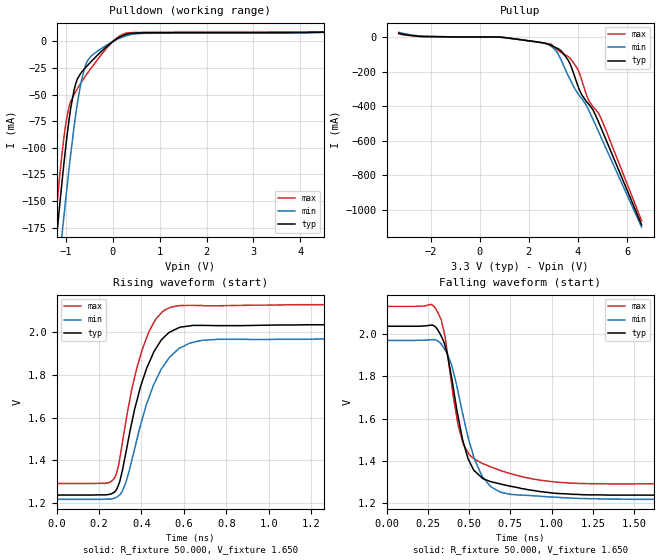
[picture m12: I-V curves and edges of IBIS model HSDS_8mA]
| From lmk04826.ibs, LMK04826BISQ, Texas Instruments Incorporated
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[Model]   HSDS_8mA
Model_type   Output
Polarity   Non-Inverting
Vmeas = 1.9
Vref = 1.9
Cref = 15pF
Rref = 50
|   typ   min   max
|   (nom PVT)   (Fast PVT)   (slow PVT)
C_comp   1.492p   1.392p   1.674p
|C_comp (hi state)   1.492p   1.392p   1.674p
|C_comp (low state)   2.777p   2.419p   2.781p
| Where   nom PVT is  Nominal Process, 3.3V, 27C
|   Fast PVT is Strong Process, 3.45V, -40C
|   Slow PVT is Weak Process, 3.15V, 125C
[Voltage Range]   3.3   3.15   3.45
[Temperature Range]   27   125   -40
[Pullup Reference]   3.3   3.15   3.45
[Pulldown Reference]   0   0   0
[Power Clamp Reference]   3.3   3.15   3.45
[GND Clamp Reference]   0   0   0
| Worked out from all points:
|   slope of the pulldown table from 0 to 0.495 V, typ, clamps not added: 61.7 ohm
|   slope of the pullup table from 0 to 0.495 V, typ, clamps not added: 8 kohm
|   falling waveform, R_fixture 50.000, V_fixture 1.650: 20-80 % time 127ps typ, 150ps min, 119ps max; typ from 2.04 V to 1.24 V
|   rising waveform, R_fixture 50.000, V_fixture 1.650: 20-80 % time 125ps typ, 142ps min, 113ps max; typ from 1.24 V to 2.04 V
[Pulldown]
|   Voltage   I(typ)   I(min)   I(max)
-3.3V     -1.226A    -1.2A      -1.253A
-1.29V    -226.6mA   -272.8mA   -200.2mA
-1.142V   -158.1mA   -207.3mA   -130.7mA
-1.082V   -131.9mA   -181.6mA   -105.5mA
-1.053V   -119.2mA   -168.9mA   -94.06mA
-973.5mV  -87.83mA   -136mA     -69.99mA
-825mV    -45.61mA   -79.95mA   -49.82mA
-686.4mV  -30.15mA   -40.74mA   -39.45mA
-607.2mV  -25.89mA   -25.84mA   -34.12mA
-409.2mV  -16.58mA   -11.85mA   -21.93mA
194.7mV   5.121mA    3.874mA    6.323mA
6.59V     10.59mA    10.66mA    10.59mA
[Pullup]
|   Voltage   I(typ)   I(min)   I(max)
-3.3V     22.42mA    27.3mA     18.86mA
-2.34V    3.185mA    4.961mA    2.641mA
897.6mV   -1.267mA   -2.718mA   -282.3uA
2.363V    -28.99mA   -28.16mA   -29.95mA
2.907V    -48.74mA   -53.27mA   -41.4mA
3.303V    -79.15mA   -129.1mA   -87.94mA
3.679V    -156.2mA   -246.1mA   -122.5mA
3.986V    -278.5mA   -324.2mA   -186mA
4.412V    -384.5mA   -415.9mA   -358.3mA
4.709V    -450mA     -507.1mA   -418.7mA
4.957V    -531.4mA   -585.3mA   -475.6mA
6.59V     -1.086A    -1.1A      -1.063A
[Ramp]
R_load = 50
|   typ   min   max
dV/dt_r   0.471953/1.25144e-10   0.443681/1.42193e-10   0.494567/1.13542e-10
dV/dt_f   0.471995/1.26586e-10   0.443829/1.50046e-10   0.494457/1.19591e-10
[Falling Waveform]
R_fixture = 50.000
V_fixture = 1.650
V_fixture_min = 1.606
V_fixture_max = 1.726
C_fixture = 0.000
|  time   V(typ)   V(min)   V(max)
0s        2.037V     1.97V      2.131V
271.7ps   2.042V     1.973V     2.14V
325.1ps   2V         1.959V     2.078V
354.5ps   1.944V     1.925V     1.989V
392.5ps   1.802V     1.859V     1.774V
466.5ps   1.485V     1.606V     1.476V
578ps     1.32V      1.329V     1.389V
699.3ps   1.289V     1.25V      1.352V
1.17ns    1.241V     1.222V     1.293V
3ns       1.238V     1.218V     1.292V
[Rising Waveform]
R_fixture = 50.000
V_fixture = 1.650
V_fixture_min = 1.606
V_fixture_max = 1.726
C_fixture = 0.000
|  time   V(typ)   V(min)   V(max)
0s        1.238V     1.218V     1.292V
271.7ps   1.251V     1.223V     1.316V
291.5ps   1.284V     1.234V     1.374V
325.1ps   1.428V     1.292V     1.573V
354.5ps   1.577V     1.4V       1.733V
405.7ps   1.776V     1.6V       1.925V
466.5ps   1.922V     1.773V     2.061V
534.2ps   2.002V     1.886V     2.117V
756.3ps   2.032V     1.968V     2.125V
3ns       2.037V     1.97V      2.131V
